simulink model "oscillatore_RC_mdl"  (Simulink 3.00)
settings: Solver=ode23s  StartTime=0.0  StopTime=10.0  RelTol=1e-6  AbsTol=1e-6
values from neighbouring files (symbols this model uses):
  beta = 60    [oscillatore.m]    (also in oscillatore_RC.m = 100; oscillatore_wien.m = 3.5)
  C = 0.001    [oscillatore.m]    (also in oscillatore_RC.m; oscillatore_RC_1.m; oscillatore_wien.m)
  K = R1/(R1+R2)    (= 0.333333333333)    [oscillatore_RC.m]    (also in oscillatore_RC_1.m)
  Q30 = C*V30    (= 0.0001)    [oscillatore.m]    (also in oscillatore_RC.m; oscillatore_RC_1.m)
  R = 1    [oscillatore.m]    (also in oscillatore_RC.m; oscillatore_RC_1.m; oscillatore_wien.m)
  tau = 0.00001    (= 1e-05)    [oscillatore.m]    (also in oscillatore_RC.m)
  VM = 12    [oscillatore.m]    (also in oscillatore_RC.m; oscillatore_RC_1.m; oscillatore_wien.m)

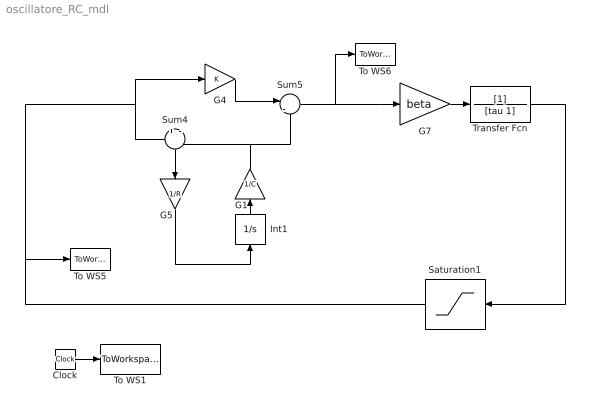
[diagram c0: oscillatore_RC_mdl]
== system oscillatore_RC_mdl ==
  Clock : Clock
  G1 : Gain  Orientation=up  Gain=1/C  SaturateOnIntegerOverflow=on
  G4 : Gain  Gain=K  SaturateOnIntegerOverflow=on
  G5 : Gain  Orientation=down  Gain=1/R  SaturateOnIntegerOverflow=on
  G7 : Gain  Gain=beta  SaturateOnIntegerOverflow=on
  Int1 : Integrator  Orientation=up  ExternalReset=none  InitialConditionSource=internal  InitialCondition=Q30  LimitOutput=off  UpperSaturationLimit=inf  LowerSaturationLimit=-inf  ShowSaturationPort=off  ShowStatePort=off  AbsoluteTolerance=auto
  Saturation1 : Saturate  Orientation=left  UpperLimit=VM  LowerLimit=-VM
  Sum4 : Sum  Orientation=down  Inputs=+|-  SaturateOnIntegerOverflow=on
  Sum5 : Sum  Inputs=+|-  SaturateOnIntegerOverflow=on
  To WS1 : ToWorkspace  VariableName=t  SampleTime=-1  SaveFormat=Matrix
  To WS5 : ToWorkspace  VariableName=V0  SampleTime=-1  SaveFormat=Matrix
  To WS6 : ToWorkspace  VariableName=VP  SampleTime=-1  SaveFormat=Matrix
  Transfer Fcn : TransferFcn  Numerator=[1]  Denominator=[tau 1]
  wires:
  Clock/1 -> To WS1/1
  Int1/1 -> G1/1
  Sum4/1 -> G5/1
  G5/1 -> Int1/1
  G1/1 -> Sum4/2, Sum5/2
  G4/1 -> Sum5/1
  Sum5/1 -> G7/1, To WS6/1
  Saturation1/1 -> To WS5/1, Sum4/1, G4/1
  G7/1 -> Transfer Fcn/1
  Transfer Fcn/1 -> Saturation1/1
